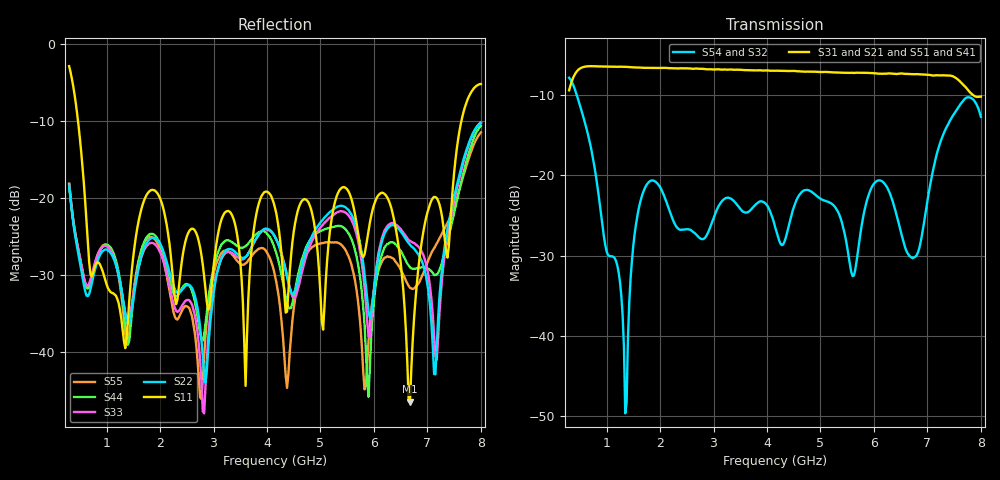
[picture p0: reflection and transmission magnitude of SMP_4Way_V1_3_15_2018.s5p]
! Created Thu Mar 15 05:36:00 2018
# hz S ma R 50
! 5 Port Network Data from SP5.SP block
! freq  magS11  angS11  magS12  angS12  magS13  angS13  magS14  angS14
!  magS15  angS15
!  magS21  angS21  magS22  angS22  magS23  angS23
!  magS24  angS24  magS25  angS25
!  magS31  angS31  magS32  angS32
!  magS33  angS33  magS34  angS34  magS35  angS35
!  magS41  angS41
!  magS42  angS42  magS43  angS43  magS44  angS44  magS45  angS45
!  magS51  angS51  magS52  angS52  magS53  angS53  magS54  angS54
!  magS55  angS55
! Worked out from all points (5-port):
!   309 points, 300 MHz to 8 GHz, reference 50 ohm
!   strongest paths, dB at 300 MHz, 2.225 GHz, 4.15 GHz, 6.075 GHz, 8 GHz:
!     S31: -9.4, -6.6, -7.0, -7.3, -10.2
!     S21: -9.4, -6.7, -7.0, -7.3, -10.1
!     S51: -9.4, -6.7, -7.0, -7.3, -10.0
!     S41: -9.4, -6.7, -7.0, -7.4, -10.2
!     S54: -7.8, -25.3, -26.4, -20.6, -12.7
!     S32: -7.8, -25.3, -26.4, -20.6, -12.7
!   lowest |S11| = -46.4 dB at 6.675 GHz (marker M1), VSWR 1.01, Z = 50.5 + j0.0417 ohm
!   |S11| at or under -10 dB: 465.3 MHz to 7.637 GHz (7.172 GHz wide, 177 % of centre)
